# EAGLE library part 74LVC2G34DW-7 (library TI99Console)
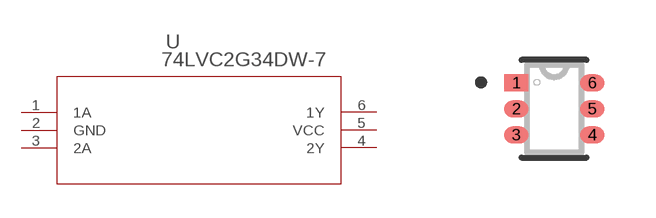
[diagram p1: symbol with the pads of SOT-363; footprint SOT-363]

Designator prefix U

## 74LVC2G34DW-7 (MANUFACTURER_PART_NUMBER: 74LVC2G34DW7; VENDOR: Diodes Inc)  [SOT-363]
1  1A  in
2  GND  pwr
3  2A  in
4  2Y  out
5  VCC  pwr
6  1Y  out

## Footprint SOT-363 (pad centres in mm)
smd 0.6 x 0.42: 1 -0.95,0.65; 2 -0.95,0; 3 -0.95,-0.65; 4 0.95,-0.65; 5 0.95,0; 6 0.95,0.65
